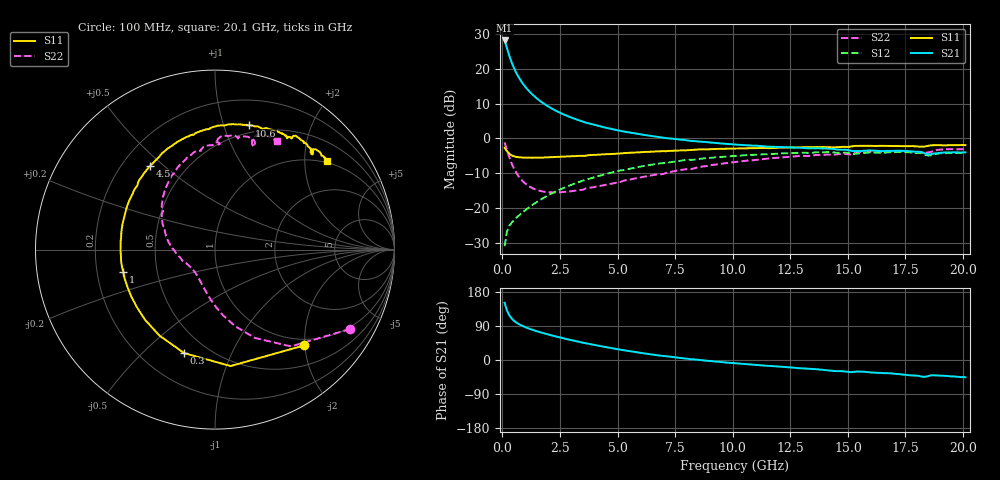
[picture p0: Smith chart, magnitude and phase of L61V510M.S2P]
!  Infineon Technologies AG
! BFR380L3 , PF131585-7, No.6, Th 09.10.01, soldered on pcb-board, measured with PP GSG850
!  Vce=1.5 V,  Ic=10.0 mA
! Common Emitter S-Parameters:  15. November 2001
#  GHz  S  MA  R  50
! f  S11  S21  S12  S22
! GHz  Mag  Ang  Mag  Ang  Mag  Ang  Mag  Ang
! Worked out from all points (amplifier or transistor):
!   201 points, 100 MHz to 20.1 GHz, reference 50 ohm
!   highest |S21| = 28.1 dB at 100 MHz (marker M1)
!   |S21| within 3 dB of that: start of sweep to 238.4 MHz
!   unconditionally stable (mu >= 1): 1.754 GHz to 4.863 GHz
!   at 3.4 GHz: K = 1.03, MAG = 7.6 dB, |S12| = -12.4 dB
!   at 10.1 GHz: K = 0.96, MSG = 1.6 dB, |S12| = -5.1 dB
!   at 20.1 GHz: K = 0.99, MSG = 0.1 dB, |S12| = -4.2 dB
!   S11 on the Smith chart (normalised r, x): 100 MHz: 0.87, -1.98; 300 MHz: 0.37, -0.68; 1 GHz: 0.31, -0.11; 4.5 GHz: 0.31, +0.45; 10.6 GHz: 0.43, +1.22; 20.1 GHz: 0.94, +2.55
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0.1  0.7284 -47.2  25.54 151.1  0.02809 67.1  0.8738 -30.4
0.2  0.6545 -82.4  19.9 130.9  0.0452 55.5  0.6856 -51.9
0.3  0.6017 -106.6  15.51 118.5  0.05478 49.8  0.5394 -65.8
0.4  0.5702 -123.0  12.48 110.0  0.06089 47.6  0.4391 -75.5
0.5  0.5522 -134.8  10.35 103.9  0.06626 47.5  0.3705 -82.8
0.6  0.5408 -143.8  8.804 99.3  0.07148 47.9  0.3221 -88.8
0.7  0.5342 -151.1  7.665 95.3  0.07647 48.8  0.2862 -93.9
0.8  0.5306 -157.0  6.77 92.0  0.08182 50.0  0.2594 -98.3
1  0.526 -166.2  5.494 86.6  0.09256 51.9  0.223 -106.0
1.2  0.5268 -173.5  4.623 82.0  0.1039 53.5  0.2005 -112.6
1.4  0.5268 -179.3  3.997 77.8  0.1155 54.6  0.1858 -118.6
1.6  0.5278 175.2  3.523 74.0  0.1276 55.5  0.1767 -123.8
1.9  0.5314 168.5  3.001 68.8  0.1459 55.9  0.1691 -130.9
2.5  0.5413 157.1  2.331 59.4  0.1833 55.3  0.1672 -142.9
3.5  0.5604 141.2  1.735 45.7  0.2465 51.8  0.1822 -158.6
4.5  0.5902 127.9  1.417 33.9  0.3074 46.7  0.2148 -173.8
6.8  0.6484 102.9  1.04 12.1  0.4331 32.0  0.3038 157.2
10.1  0.712 77.7  0.8124 -8.7  0.5576 10.7  0.4559 125.1
10.6  0.718 74.5  0.7915 -11.1  0.5722 7.5  0.4773 120.4
13.5  0.7458 59.9  0.7199 -23.6  0.623 -10.1  0.5669 97.4
16.8  0.7731 47.8  0.6596 -34.9  0.6267 -25.9  0.6492 76.4
20.1  0.7964 38.5  0.628 -45.5  0.619 -39.4  0.6994 60.3
